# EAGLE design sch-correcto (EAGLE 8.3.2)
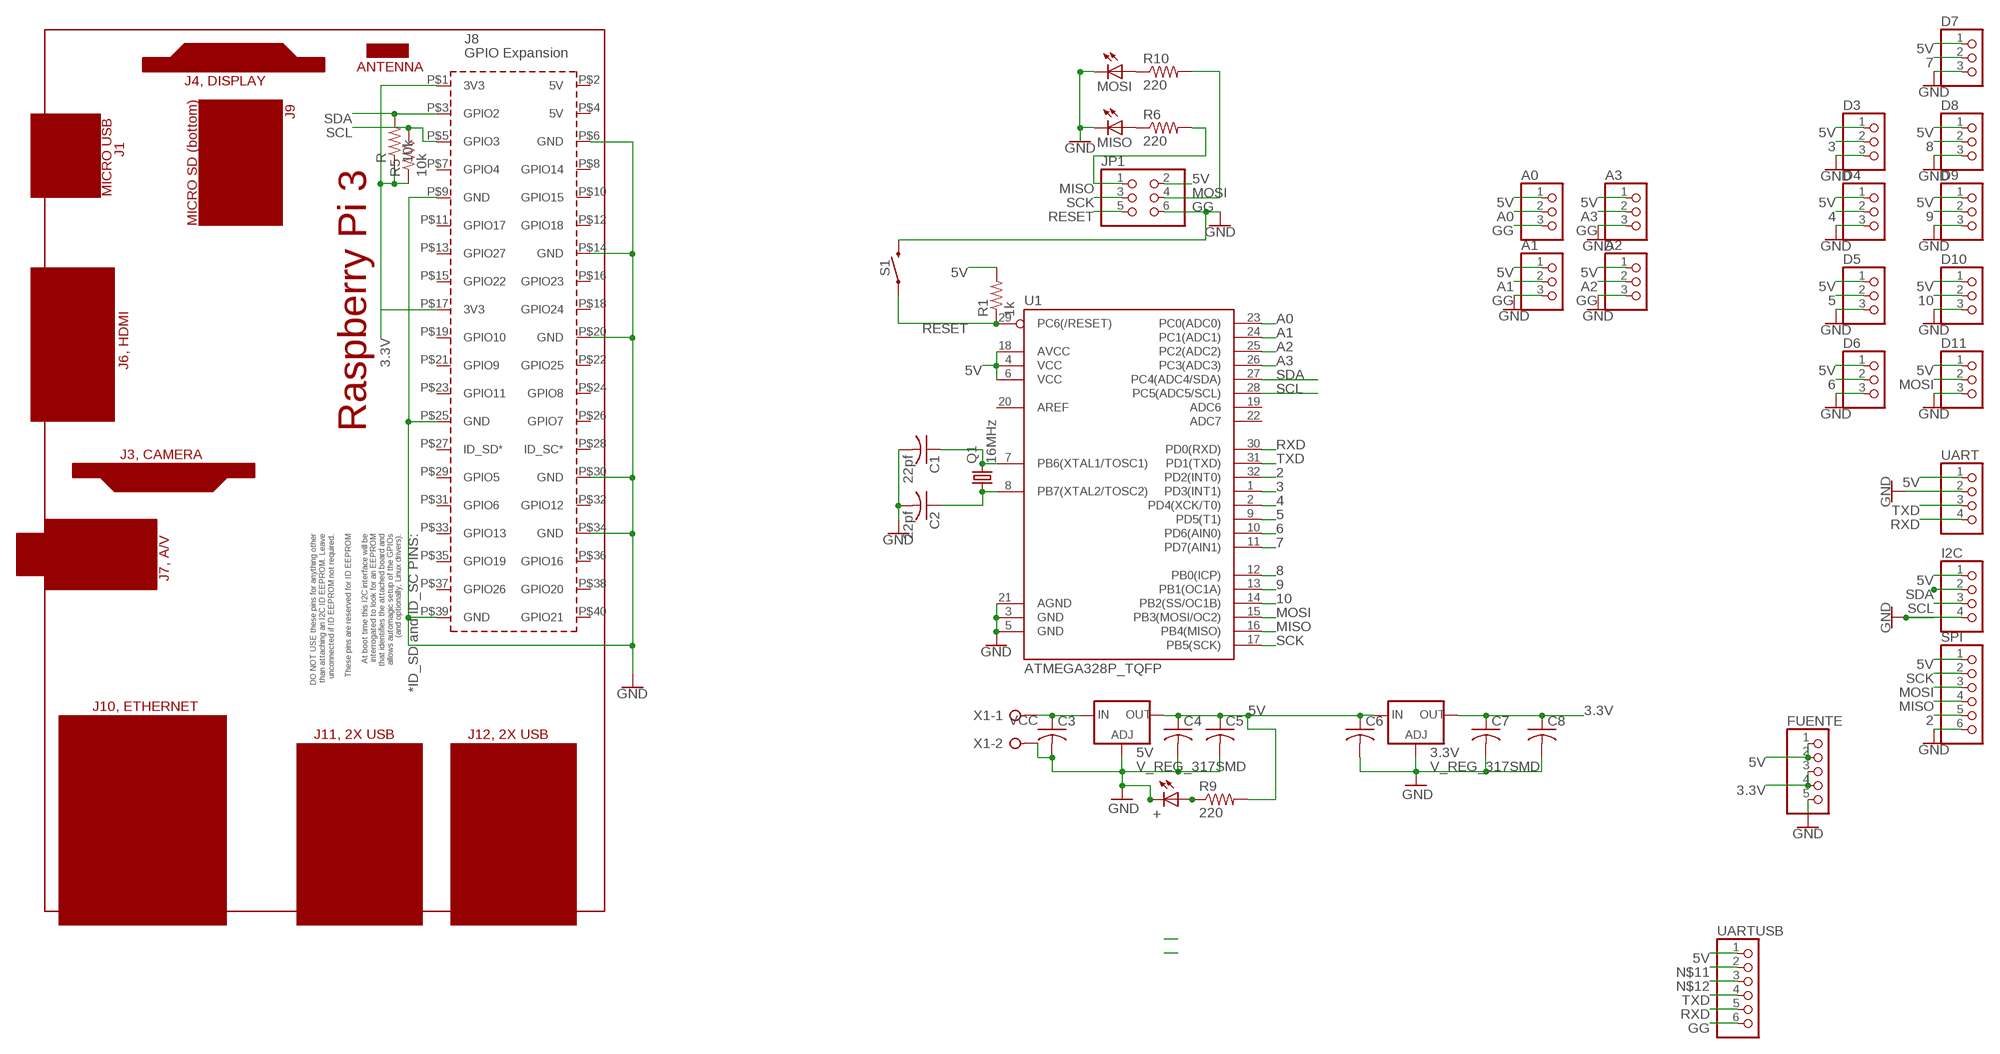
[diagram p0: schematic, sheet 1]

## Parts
3.3V  V_REG_317SMD  [SOT223]
5V  V_REG_317SMD  [SOT223]
+  LEDSML1206  [SML1206]
A0  PINHD-1X3  [1X03]
A1  PINHD-1X3  [1X03]
A2  PINHD-1X3  [1X03]
A3  PINHD-1X3  [1X03]
C1  22pf  C-USC1206  [C1206]
C2  22pf  C-USC1206  [C1206]
C3  C-USC1206  [C1206]
C4  C-USC1206  [C1206]
C5  C-USC1206  [C1206]
C6  C-USC1206  [C1206]
C7  C-USC1206  [C1206]
C8  C-USC1206  [C1206]
D3  PINHD-1X3  [1X03]
D4  PINHD-1X3  [1X03]
D5  PINHD-1X3  [1X03]
D6  PINHD-1X3  [1X03]
D7  PINHD-1X3  [1X03]
D8  PINHD-1X3  [1X03]
D9  PINHD-1X3  [1X03]
D10  PINHD-1X3  [1X03]
D11  PINHD-1X3  [1X03]
FUENTE  PINHD-1X5  [1X05]
I2C  PINHD-1X4  [1X04]
JP1  PINHD-2X3  [2X03]
MISO  LEDSML1206  [SML1206]
MOSI  LEDSML1206  [SML1206]
PCB1  RPI3  [RPI3]
Q1  16MHz  CRYSTALHC49UP  [HC49UP]
R  10k  R-US_M1206  [M1206]
R1  1k  R-US_M1206  [M1206]
R5  10k  R-US_M1206  [M1206]
R6  220  R-US_M1206  [M1206]
R9  220  R-US_M1206  [M1206]
R10  220  R-US_M1206  [M1206]
S1  MOMENTARY-SWITCH-SPST-SMD-6.2MM-TALL  [TACTILE_SWITCH_SMD_6.2MM_TALL]
SPI  PINHD-1X6  [1X06]
U1  ATMEGA328P_TQFP  [TQFP32-08]
UART  PINHD-1X4  [1X04]
UARTUSB  PINHD-1X6  [1X06]
X1  W237-02P  [W237-132]

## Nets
2: SPI.5 U1.32(PD2(INT0))
3: D3.2 U1.1(PD3(INT1))
3.3V: 3.3V.2(OUT) C7.1 C8.1 FUENTE.3 FUENTE.4 PCB1.P$1(3V3) PCB1.P$17(3V3) R5.1 R.1
4: D4.2 U1.2(PD4(XCK/T0))
5: D5.2 U1.9(PD5(T1))
5V: 3.3V.3(IN) 5V.2(OUT) A0.1 A1.1 A2.1 A3.1 C4.1 C5.1 C6.1 D3.1 D4.1 D5.1 D6.1 D7.1 D8.1 D9.1 D10.1 D11.1 FUENTE.1 FUENTE.2 I2C.1 JP1.2 R1.2 R9.2 SPI.1 U1.4(VCC) U1.6(VCC) U1.18(AVCC) UART.1 UARTUSB.1
6: D6.2 U1.10(PD6(AIN0))
7: D7.2 U1.11(PD7(AIN1))
8: D8.2 U1.12(PB0(ICP))
9: D9.2 U1.13(PB1(OC1A))
10: D10.2 U1.14(PB2(SS/OC1B))
A0: A0.2 U1.23(PC0(ADC0))
A1: A1.2 U1.24(PC1(ADC1))
A2: A2.2 U1.25(PC2(ADC2))
A3: A3.2 U1.26(PC3(ADC3))
GG: 3.3V.1(ADJ) 5V.1(ADJ) +.C A0.3 A1.3 A2.3 A3.3 C1.2 C2.2 C3.2 C4.2 C5.2 C6.2 C7.2 C8.2 D3.3 D4.3 D5.3 D6.3 D7.3 D8.3 D9.3 D10.3 D11.3 FUENTE.5 I2C.4 JP1.6 MISO.C MOSI.C PCB1.P$6(GND) PCB1.P$9(GND) PCB1.P$14(GND) PCB1.P$20(GND) PCB1.P$25(GND) PCB1.P$30(GND) PCB1.P$34(GND) PCB1.P$39(GND) S1.B2 SPI.6 U1.3(GND) U1.5(GND) U1.21(AGND) UART.2 UARTUSB.6 X1.2 ; supply symbol labelled GND
MISO: JP1.1 R6.2 SPI.4 U1.16(PB4(MISO))
MOSI: D11.2 JP1.4 R10.2 SPI.3 U1.15(PB3(MOSI/OC2))
N$1: C1.1 Q1.2 U1.7(PB6(XTAL1/TOSC1))
N$2: C2.1 Q1.1 U1.8(PB7(XTAL2/TOSC2))
N$4: +.A R9.1
N$8: MISO.A R6.1
N$9: MOSI.A R10.1
N$11: UARTUSB.2
N$12: UARTUSB.3
RESET: JP1.5 R1.1 S1.A2 U1.29(PC6(/RESET))
RXD: U1.30(PD0(RXD)) UART.4 UARTUSB.5
SCK: JP1.3 SPI.2 U1.17(PB5(SCK))
SCL: I2C.3 PCB1.P$5(GPIO3) R5.2 U1.28(PC5(ADC5/SCL))
SDA: I2C.2 PCB1.P$3(GPIO2) R.2 U1.27(PC4(ADC4/SDA))
TXD: U1.31(PD1(TXD)) UART.3 UARTUSB.4
VCC: 5V.3(IN) C3.1 X1.1
Unconnected: PCB1.P$2(5V) PCB1.P$4(5V) PCB1.P$7(GPIO4) PCB1.P$8(GPIO14) PCB1.P$10(GPIO15) PCB1.P$11(GPIO17) PCB1.P$12(GPIO18) PCB1.P$13(GPIO27) PCB1.P$15(GPIO22) PCB1.P$16(GPIO23) PCB1.P$18(GPIO24) PCB1.P$19(GPIO10) PCB1.P$21(GPIO9) PCB1.P$22(GPIO25) PCB1.P$23(GPIO11) PCB1.P$24(GPIO8) PCB1.P$26(GPIO7) PCB1.P$27(ID_SD*) PCB1.P$28(ID_SC*) PCB1.P$29(GPIO5) PCB1.P$31(GPIO6) PCB1.P$32(GPIO12) PCB1.P$33(GPIO13) PCB1.P$35(GPIO19) PCB1.P$36(GPIO16) PCB1.P$37(GPIO26) PCB1.P$38(GPIO20) PCB1.P$40(GPIO21) U1.19(ADC6) U1.20(AREF) U1.22(ADC7)

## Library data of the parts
3.3V 5V = SparkFun-IC-Power:V_REG_317: Voltage Regulator Standard LM317 adjustable voltage regulator. AOI (Adjust Output Input). Google 'LM317 Calculator' for easy to use app to get the two resistor values needed. 240/720 for 5V output. 240/390 for 3.3V output. Spark Fun Electronics SKU : COM-00527
+ MISO MOSI = led:LED: LED
A0 A1-A3 D3-D11 = pinhead:PINHD-1X3: PIN HEADER
C1 C2 = rcl:C-US: CAPACITOR, American symbol
C3-C8 = resistor:C-US: CAPACITOR, American symbol
FUENTE = pinhead:PINHD-1X5: PIN HEADER
I2C UART = pinhead:PINHD-1X4: PIN HEADER
JP1 = pinhead:PINHD-2X3: PIN HEADER
PCB1 = e14_Rpi3_RevA:RPI3: Device for Raspberry Pi 3 board created by Dave Young for www.element14.com More information and support community is available at https://www.element14.com/community/community/raspberry-pi
Q1 = crystal:CRYSTAL: CRYSTAL; OC_FARNELL: unknown; OC_NEWARK: unknown
R R1 R5 R6 R9 R10 = resistor:R-US_: RESISTOR, American symbol
S1 = SparkFun-Switches:MOMENTARY-SWITCH-SPST: Momentary Switch (Pushbutton) - SPST; PROD_ID: SWCH-11966; SF_SKU: COM-12992
SPI UARTUSB = pinhead:PINHD-1X6: PIN HEADER
U1 = SparkFun-DigitalIC:ATMEGA328P_TQFP; PROD_ID: IC-09069
X1 = con-wago-508:W237-02P: WAGO SREW CLAMP; OC_FARNELL: unknown; OC_NEWARK: unknown

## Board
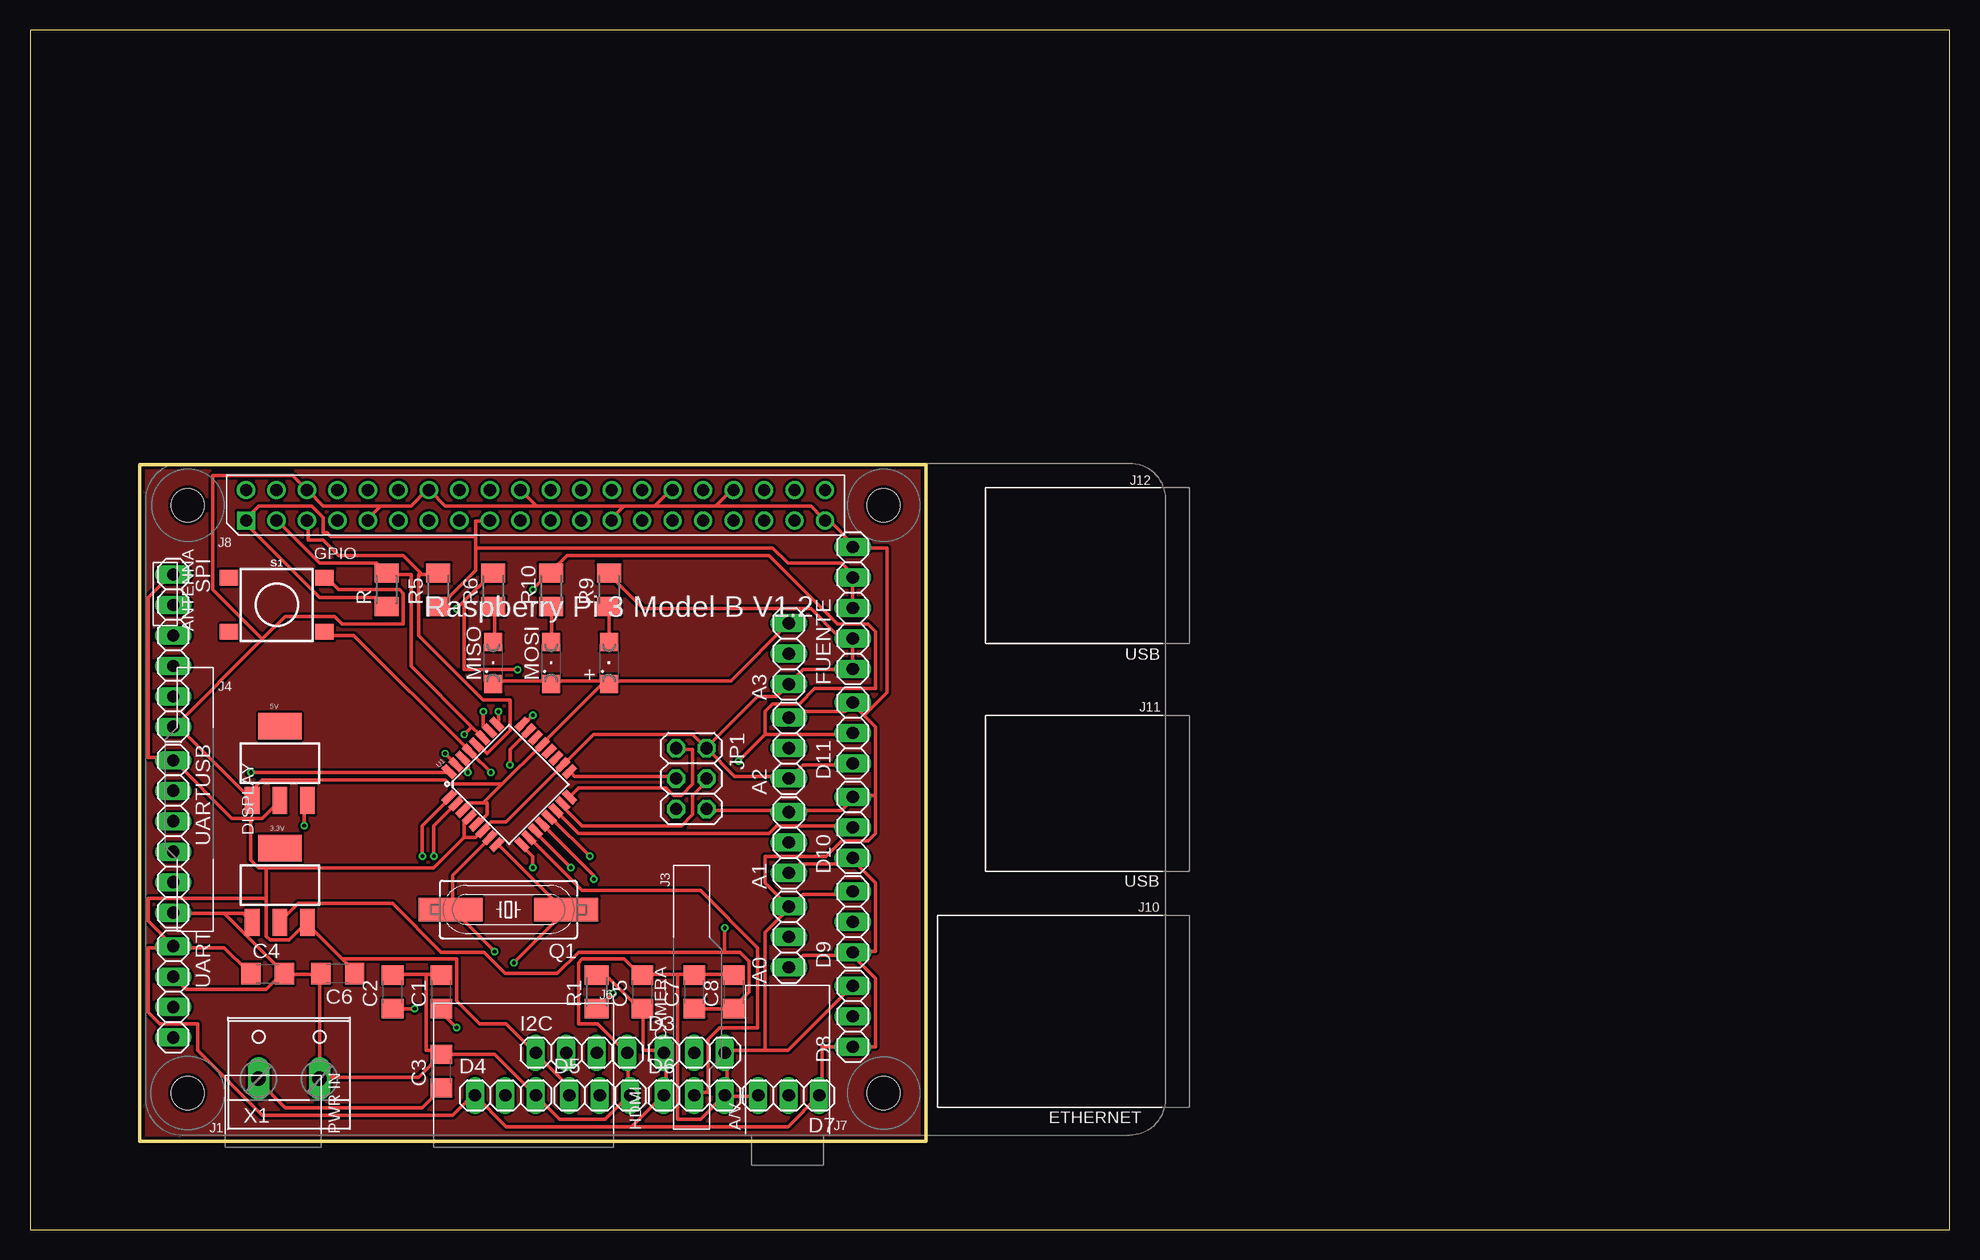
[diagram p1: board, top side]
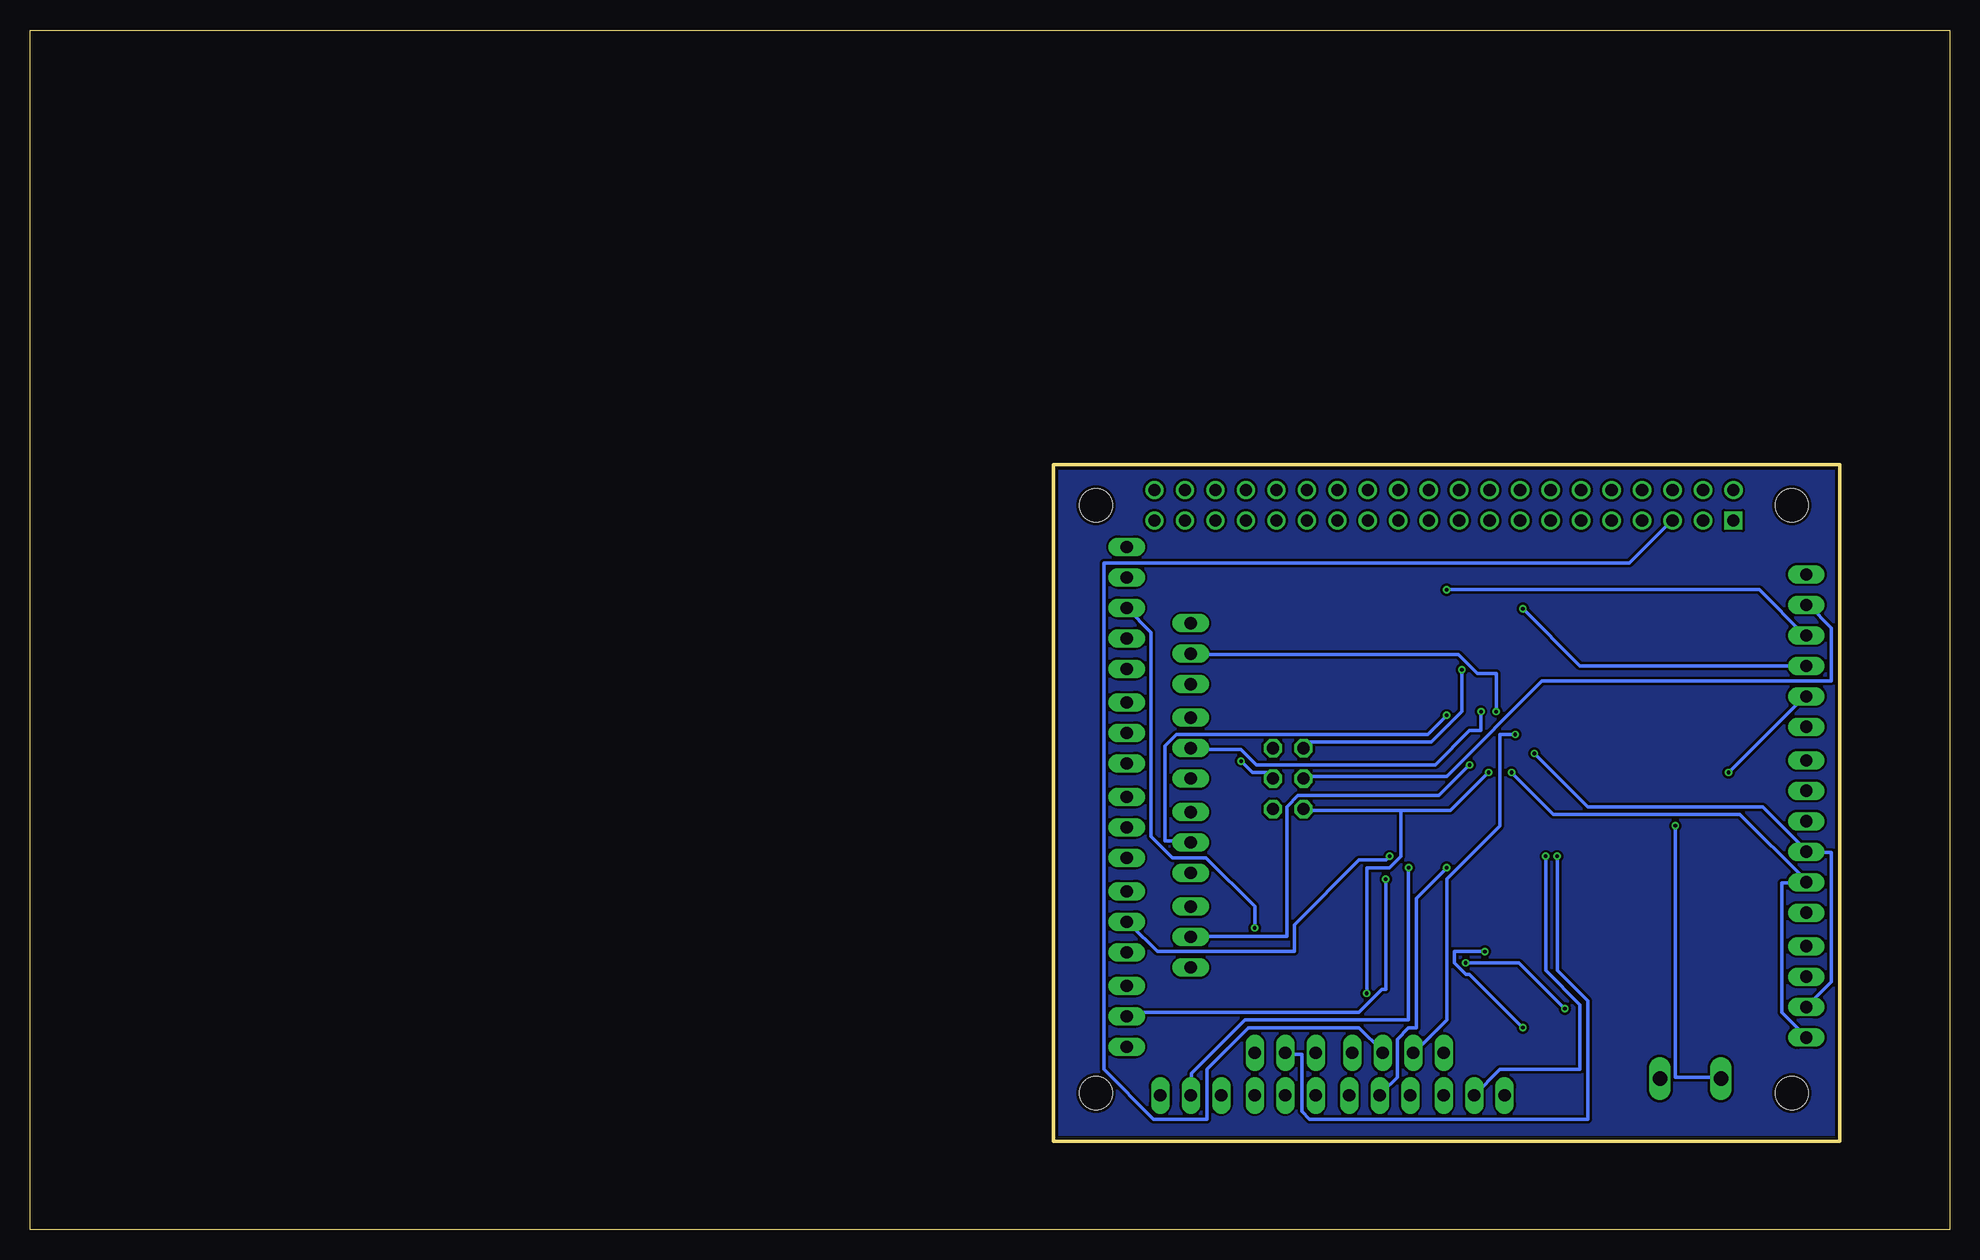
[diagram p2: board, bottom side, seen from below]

Size 160 x 100 mm. Coordinates in mm from the lower left corner, seen from the top.
Outline: 0,0 160,0 160,100 0,100 0,0
Outline: 9.14,7.37 74.68,7.37 74.68,63.75 9.14,63.75 9.14,7.37
Copper layers (1*16): Top 0.035mm / dielectric 1.5mm / Bottom 0.035mm
Design rules "RYSPEE_2layer_DRU *": minimum track width 12mil, minimum drill 12mil, track to track 8mil, track to pad 8mil, pad to pad 8mil, via to via 8mil, smd to smd 8mil, copper to edge 10mil, drill to drill 10mil, minimum pad ring 10mil, minimum via ring 6mil, stop-mask expansion 2mil, vias tented up to drill 100mil, thermal gap 10mil

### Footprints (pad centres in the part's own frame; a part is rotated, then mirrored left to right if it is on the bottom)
SOT223 = smd 1.219 x 2.235: 1 -2.311,-3.099; 2 0,-3.099; 3 2.311,-3.099 | smd 3.6 x 2.2: 4 0,3.099
SML1206 = smd 1.5 x 1.5: A 1.75,0; C -1.75,0
1X03 = drill 1.016 long: 1 -2.54,0; 2 0,0; 3 2.54,0
C1206 = smd 1.6 x 1.8: 1 -1.4,0; 2 1.4,0
1X05 = drill 1.016 long: 1 -5.08,0; 2 -2.54,0; 3 0,0; 4 2.54,0; 5 5.08,0
1X04 = drill 1.016 long: 1 -3.81,0; 2 -1.27,0; 3 1.27,0; 4 3.81,0
2X03 = drill 1.016 octagon: 1 -2.54,-1.27; 2 -2.54,1.27; 3 0,-1.27; 4 0,1.27; 5 2.54,-1.27; 6 2.54,1.27
RPI3 = drill 1.016 square: P$1 8.37,51.23 | drill 1.016: P$2 8.357,53.772; P$3 10.897,51.232; P$4 10.897,53.772; P$5 13.437,51.232; P$6 13.437,53.772; P$7 15.977,51.232; P$8 15.977,53.772; P$9 18.517,51.232; P$10 18.517,53.772; P$11 21.057,51.232; P$12 21.057,53.772; P$13 23.597,51.232; P$14 23.597,53.772; P$15 26.137,51.232; P$16 26.137,53.772; P$17 28.677,51.232; P$18 28.677,53.772; P$19 31.217,51.232; P$20 31.217,53.772; P$21 33.757,51.232; P$22 33.757,53.772; P$23 36.297,51.232; P$24 36.297,53.772; P$25 38.837,51.232; P$26 38.837,53.772; P$27 41.377,51.232; P$28 41.377,53.772; P$29 43.917,51.232; P$30 43.917,53.772; P$31 46.457,51.232; P$32 46.457,53.772; P$33 48.997,51.232; P$34 48.997,53.772; P$35 51.537,51.232; P$36 51.537,53.772; P$37 54.077,51.232; P$38 54.077,53.772; P$39 56.617,51.232; P$40 56.617,53.772 | hole 2.75: 3.5,3.5; 61.5,3.5; 3.5,52.5; 61.5,52.5
HC49UP = smd 5.334 x 1.93: 1 -4.826,0; 2 4.826,0
M1206 = smd 1.6 x 2: 1 -1.4,0; 2 1.4,0
TACTILE_SWITCH_SMD_6.2MM_TALL = smd 1.55 x 1.3: A1 -3.975,-2.25; A2 3.975,-2.25; B1 -3.975,2.25; B2 3.975,2.25
1X06 = drill 1.016 long: 1 -6.35,0; 2 -3.81,0; 3 -1.27,0; 4 1.27,0; 5 3.81,0; 6 6.35,0
TQFP32-08 = smd 1.27 x 0.559: 1 -4.293,2.8; 2 -4.293,2; 3 -4.293,1.2; 4 -4.293,0.4; 5 -4.293,-0.4; 6 -4.293,-1.2; 7 -4.293,-2; 8 -4.293,-2.8; 17 4.293,-2.8; 18 4.293,-2; 19 4.293,-1.2; 20 4.293,-0.4; 21 4.293,0.4; 22 4.293,1.2; 23 4.293,2; 24 4.293,2.8 | smd 0.559 x 1.27: 9 -2.8,-4.293; 10 -2,-4.293; 11 -1.2,-4.293; 12 -0.4,-4.293; 13 0.4,-4.293; 14 1.2,-4.293; 15 2,-4.293; 16 2.8,-4.293; 25 2.8,4.293; 26 2,4.293; 27 1.2,4.293; 28 0.4,4.293; 29 -0.4,4.293; 30 -1.2,4.293; 31 -2,4.293; 32 -2.8,4.293
W237-132 = drill 1.194 long: 1 -2.54,-0.635; 2 2.54,-0.635

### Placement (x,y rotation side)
3.3V  20.83,28.7 0 top
5V  20.83,38.86 0 top
+  48.26,47.24 90 top
A0  63.25,24.38 90 top
A1  63.25,32.26 90 top
A2  63.25,40.13 90 top
A3  63.25,48.01 90 top
C1  34.29,19.81 90 top
C2  30.23,19.81 90 top
C3  34.29,13.21 90 top
C4  19.81,21.34 0 top
C5  51.05,19.81 90 top
C6  25.65,21.34 180 top
C7  55.37,19.81 90 top
C8  58.67,19.81 90 top
D3  55.37,14.73 0 top
D4  39.62,11.18 0 top
D5  47.5,11.18 0 top
D6  55.37,11.18 0 top
D7  63.25,11.18 180 top
D8  68.58,17.78 90 top
D9  68.58,25.65 90 top
D10  68.58,33.53 90 top
D11  68.58,41.4 90 top
FUENTE  68.58,51.82 90 top
I2C  45.97,14.73 0 top
JP1  55.12,37.59 270 top
MISO  38.61,47.24 90 top
MOSI  43.43,47.24 90 top
PCB1  9.65,7.87 0 top
Q1  39.88,26.67 180 top
R  29.72,53.34 90 top
R1  47.24,19.81 90 top
R5  34.04,53.34 90 top
R6  38.61,53.34 90 top
R9  48.26,53.34 90 top
R10  43.43,53.34 90 top
S1  20.57,52.07 0 top
SPI  11.94,48.26 270 top
U1  39.95,37.11 45 top
UART  11.94,19.81 270 top
UARTUSB  11.94,32.77 270 top
X1  21.59,13.21 0 top

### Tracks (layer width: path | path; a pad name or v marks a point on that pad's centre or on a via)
2  (via drill 0.3)
  Top 0.305: v18.41,38.1 34.92,38.1 U1.32
  Bottom 0.305: v18.41,38.1 12.06,44.45 SPI.5
3  (via drill 0.3)
  Top 0.305: v32.7,31.11 32.7,33.66 34.92,35.88 U1.1
  Bottom 0.305: v32.7,31.11 32.7,21.59 30.16,19.05 30.16,9.21 53.34,9.21 53.98,9.84 53.98,14.61 55.24,14.61 D3.2
3.3V  (via drill 0.3)
  Top 0.305: C7.1 55.56,18.41 58.42,18.41 C8.1 58.67,18.54 59.94,19.81 59.94,22.35 59.18,23.11 57.91,23.11 | R.1 29.53,52.07 28.89,52.7 24.13,52.7 17.78,59.05 PCB1.P$1 18.1,59.37 19.05,60.33 23.5,60.33 24.45,59.37 24.45,58.1 24.77,58.1 25.08,57.78 37.15,57.78 | FUENTE.3 FUENTE.4 68.58,54.61 67.63,55.56 63.18,55.56 61.91,56.83 37.15,56.83 | 37.15,57.78 37.15,59.05 38.1,59.05 PCB1.P$17 | 37.15,57.78 37.15,56.83 | 37.15,56.83 37.15,54.93 34.29,52.07 R5.1 | 57.91,23.11 45.72,23.11 43.94,21.34 39.62,21.34 37.85,23.11 34.29,23.11 30.23,27.18 22.35,27.18 20.83,25.65 3.3V.2 | v57.91,25.15 57.91,23.11
  Bottom 0.305: v57.91,25.15 57.91,26.92 61.98,30.99 64.77,30.99 66.55,32.77 66.55,49.78 FUENTE.3
4  (via drill 0.3)
  Top 0.305: v33.66,31.11 33.66,33.66 35.24,35.24 U1.2
  Bottom 0.305: v33.66,31.11 33.66,21.59 30.8,18.73 30.8,13.34 37.47,13.34 D4.2
5  (via drill 0.3)
  Top 0.305: v41.91,30.16 41.91,31.11 40.96,32.07 U1.9
  Bottom 0.305: v41.91,30.16 44.45,27.62 44.45,16.83 45.09,16.83 46.04,15.88 46.04,12.7 47.31,11.43 D5.2
5V
  Top 0.305: 68.58,30.8 68.26,30.48 64.14,30.48 63.5,29.84 A1.1 | 68.58,22.86 64.45,22.86 63.5,21.91 A0.1 | 68.58,22.86 70.48,20.95 70.48,15.24 D8.1 66.04,15.24 66.04,11.43 D7.1 63.18,8.57 50.16,8.57 | 68.58,22.86 D9.1 68.58,23.18 70.48,23.18 70.48,28.89 68.58,30.8 | 68.58,30.8 D10.1 | R1.2 47.31,20.95 48.26,20.95 50.8,18.41 C5.1 51.12,18.1 51.12,14.92 52.7,14.92 D3.1 53.02,14.61 53.02,11.43 D6.1 52.7,11.11 50.16,8.57 | 50.16,8.57 39.69,8.57 D4.1 36.83,11.11 35.24,9.53 19.37,9.53 13.97,14.92 13.97,17.14 10.79,17.14 9.84,18.1 9.84,23.5 11.75,23.5 UART.1 | R9.2 48.26,54.61 51.12,51.75 65.09,51.75 67.31,49.53 68.58,49.53 FUENTE.2 FUENTE.1 68.58,46.67 64.45,46.67 A3.1 62.23,44.45 60.64,44.45 56.52,40.32 JP1.2 | 36.2,32.7 36.2,33.97 36.51,34.29 U1.4 | 36.2,32.7 37.15,32.7 37.47,33.02 U1.6 37.78,33.34 38.42,33.97 39.69,33.97 44.45,38.73 | D11.1 68.58,38.73 64.45,38.73 63.5,37.78 A2.1 63.18,37.78 58.74,37.78 JP1.2 | 44.45,38.73 46.99,41.27 55.24,41.27 JP1.2 | 44.45,38.73 U1.18 | C4.1 18.1,21.59 16.19,23.5 12.06,23.5 UART.1 | D5.1 44.77,11.43 44.77,12.06 42.23,14.61 I2C.1 41.91,14.92 39.69,17.14 37.47,17.14 35.56,19.05 35.56,22.54 26.04,22.54 | 26.04,22.54 23.18,25.4 3.3V.3 22.86,25.4 21.59,24.13 20,24.13 19.68,24.45 19.68,27.62 | 26.04,22.54 26.99,21.59 C6.1 | 18.41,34.29 16.83,34.29 12.06,39.05 UARTUSB.1 11.75,39.37 9.84,39.37 9.84,52.7 11.75,54.61 SPI.1 | 18.41,34.29 19.37,34.29 20.64,35.56 5V.2 | 19.68,30.16 19.68,27.62 | 19.68,30.16 19.05,30.16 18.41,30.8 18.41,34.29 | UART.1 9.84,25.72 9.84,27.62 19.68,27.62 | 36.2,32.7 33.66,30.16 19.68,30.16
6
  Top 0.305: U1.10 41.59,32.7 46.04,28.26 55.88,28.26 60.64,23.5 60.64,16.83 57.47,16.83 56.52,15.88 56.52,11.43 55.56,11.43 D6.2
7  (via drill 0.3)
  Top 0.305: v45.09,30.16 42.23,33.02 U1.11
  Bottom 0.305: v45.09,30.16 45.09,17.46 58.74,17.46 63.18,13.02 63.18,11.43 D7.2
8  (via drill 0.3)
  Top 0.305: v46.99,29.21 46.99,29.53 42.86,33.66 U1.12
  Bottom 0.305: v46.99,29.21 46.99,20 47.31,20 49.21,18.1 68.26,18.1 D8.2
9  (via drill 0.3)
  Top 0.305: v46.67,31.11 43.5,34.29 U1.13
  Bottom 0.305: v46.67,31.11 46.99,30.8 49.21,30.8 54.61,25.4 54.61,23.18 66.04,23.18 68.26,25.4 68.58,25.4 D9.2
10
  Top 0.305: U1.14 43.81,34.92 45.72,33.02 61.59,33.02 62.23,33.66 68.58,33.66 D10.2
A0  (via drill 0.3)
  Top 0.305: v40.01,38.73 40.01,40.01 41.27,41.27 U1.23
  Bottom 0.305: v40.01,38.73 42.55,36.2 54.29,36.2 55.24,35.24 55.24,24.45 63.18,24.45 A0.2
A1  (via drill 0.3)
  Top 0.305: v41.91,42.86 41.27,42.23 U1.24
  Bottom 0.305: v41.91,42.86 43.5,41.27 64.45,41.27 65.41,40.32 65.41,32.38 63.5,32.38 A1.2
A2  (via drill 0.3)
  Top 0.305: v39.05,43.18 39.05,42.23 U1.25
  Bottom 0.305: v39.05,43.18 39.05,41.59 40.01,41.59 42.86,38.73 57.78,38.73 59.05,40.01 63.18,40.01 A2.2
A3  (via drill 0.3)
  Top 0.305: v37.78,43.18 37.78,41.91 38.1,41.59 U1.26
  Bottom 0.305: v37.78,43.18 37.78,46.35 39.37,46.35 40.96,47.94 63.18,47.94 A3.2
GG
  Top 0.305: A0.3 63.5,26.99 64.45,27.94 68.58,27.94 D9.3 | 53.98,21.27 55.24,21.27 C7.2 55.56,21.27 58.42,21.27 C8.2 | 53.98,21.27 51.12,21.27 C5.2 50.8,21.27 49.53,22.54 46.04,22.54 45.72,22.23 45.72,17.14 47.31,17.14 49.53,14.92 I2C.4 49.85,14.61 49.85,11.43 D5.3 49.85,11.11 47.94,9.21 44.13,9.21 D4.3 38.73,14.61 C3.2 | D6.3 58.1,11.11 60.64,11.11 D7.3 | D6.3 58.1,11.43 58.1,14.61 D3.3 58.1,14.92 61.28,14.92 | D8.3 63.18,14.92 61.28,14.92 | 53.98,21.27 53.98,9.21 55.88,9.21 57.78,11.11 D6.3 | 61.28,14.92 61.28,24.77 63.18,26.67 A0.3 | 24.13,21.27 21.27,21.27 C4.2 | 16.19,26.35 12.06,26.35 UARTUSB.6 | 16.19,26.35 17.78,26.35 18.41,25.72 3.3V.1 | 16.19,26.35 20.95,21.59 C4.2 | UART.2 13.02,20 19.68,20 20.95,21.27 C4.2 | 33.02,21.27 34.29,21.27 C1.2 | 33.02,21.27 30.48,21.27 C2.2 | C3.2 32.38,12.7 24.13,12.7 | C3.2 34.29,14.92 33.02,14.92 33.02,21.27 | 24.13,12.7 24.13,21.27 | 24.13,21.27 C6.2 | 24.13,12.7 X1.2 | 12.06,41.91 19.37,49.21 | 19.37,49.21 21.27,51.12 25.4,51.12 26.04,50.48 31.11,50.48 31.11,53.02 30.8,53.34 25.72,53.34 24.77,54.29 S1.B2 | 18.1,36.2 12.38,41.91 12.06,41.91 | 18.1,36.2 18.41,35.88 5V.1 18.1,36.2 | 12.06,41.91 SPI.6 | 37.78,35.56 36.51,35.56 36.2,35.24 U1.3 | 37.78,35.56 38.1,35.56 38.1,34.61 37.47,33.97 U1.5 | 37.78,35.56 39.37,37.15 | 39.37,37.15 42.55,40.32 U1.21 42.86,40.64 47.94,45.72 | MISO.C 38.73,45.72 43.18,45.72 MOSI.C 43.5,45.72 47.94,45.72 | 47.94,45.72 48.26,45.72 | A3.3 58.42,45.72 48.26,45.72 | 48.26,45.72 +.C 47.94,45.72 | 18.1,36.2 19.37,37.47 34.61,37.47 34.92,37.15 39.37,37.15 | 68.58,43.81 67.94,43.18 63.82,43.18 63.5,42.86 A2.3 | JP1.6 56.52,34.92 63.18,34.92 A1.3 63.5,34.92 67.63,34.92 68.58,35.88 D10.3 68.58,36.2 70.48,36.2
  Top 0.305: 69.53,42.86 70.48,41.91 70.48,36.2 | 69.53,42.86 68.58,43.81 | 68.58,43.81 D11.3 | 29.21,60.33 28.26,59.37 PCB1.P$9 | 29.21,60.33 31.75,60.33 33.02,61.59 PCB1.P$14 33.34,61.59 34.61,60.33 42.23,60.33 | 29.21,60.33 24.45,60.33 23.18,61.59 PCB1.P$6 22.86,61.91 21.91,62.87 15.24,62.87 15.24,53.34 19.37,49.21 | 49.53,60.33 48.58,59.37 PCB1.P$25 | 52.07,60.33 49.53,60.33 | 52.07,60.33 53.34,61.59 PCB1.P$30 | 42.23,60.33 40.96,61.59 PCB1.P$20 | 49.53,60.33 42.23,60.33 | 57.15,60.33 58.42,61.59 PCB1.P$34 | 52.07,60.33 57.15,60.33 | 57.15,60.33 65.09,60.33 66.04,59.37 PCB1.P$39 66.36,59.05 66.67,59.05 68.58,57.15 FUENTE.5 68.58,56.83 71.44,56.83 71.44,44.77 69.53,42.86 | A0.3 61.28,28.89 61.28,31.11 66.36,31.11 67.63,32.38 69.85,32.38 70.48,33.02 70.48,36.2
GND
  pour Top: 9.4,7.62 74.42,7.62 74.42,63.5 9.4,63.5
  pour Bottom: 9.4,7.62 74.42,7.62 74.42,63.5 9.4,63.5
MISO  (via drill 0.3)
  Top 0.305: U1.16 45.09,36.2 45.72,36.83 53.02,36.83 53.66,36.2 54.29,36.2 55.24,37.15 55.24,40.01 53.98,40.01 JP1.1 | v35.56,51.75 36.2,52.39 | 36.2,52.39 38.42,54.61 R6.2 | v40.64,46.67 36.2,46.67 36.2,52.39
  Bottom 0.305: v35.56,51.75 30.8,46.99 SPI.4 | JP1.1 53.34,40.64 43.18,40.64 40.64,43.18 v40.64,46.67
MOSI  (via drill 0.3)
  Top 0.305: U1.15 44.45,35.24 46.04,33.66 54.29,33.66 55.24,34.61 55.24,36.2 56.52,37.47 JP1.4 | 61.28,41.27 61.28,43.18 61.91,43.81 64.14,43.81 65.41,45.09 70.48,45.09 70.48,49.85 69.85,50.48 67.31,50.48 61.59,56.2 44.77,56.2 43.5,54.93 R10.2 43.18,54.61 v41.91,53.34 | 61.28,41.27 68.58,41.27 D11.2 | 61.28,41.27 v59.05,39.05
  Bottom 0.305: v41.91,53.34 15.88,53.34 12.06,49.53 SPI.3 | v59.05,39.05 58.1,38.1 56.83,38.1 56.52,37.78 JP1.4
N$1  (via drill 0.3)
  Top 0.305: 35.24,26.67 35.24,29.53 38.1,32.38 U1.7 | v35.56,16.83 34.29,18.1 C1.1 | 35.24,26.67 v38.73,23.18 | 35.24,26.67 Q1.2
  Bottom 0.305: v35.56,16.83 40.01,21.27 40.32,21.27 41.27,22.23 41.27,23.18 v38.73,23.18
N$2  (via drill 0.3)
  Top 0.305: 44.45,26.67 39.05,32.07 U1.8 | v32.07,18.41 30.48,18.41 C2.1 | v40.32,22.23 44.45,26.35 44.45,26.67 | 44.45,26.67 Q1.1
  Bottom 0.305: v32.07,18.41 35.88,22.23 v40.32,22.23
N$4
  Top 0.305: R9.1 +.A
N$8
  Top 0.305: MISO.A 38.73,49.21 38.73,51.75 R6.1
N$9
  Top 0.305: MOSI.A 43.5,49.21 43.5,51.75 R10.1
RESET  (via drill 0.3)
  Top 0.305: S1.A2 24.77,49.53 26.99,49.53 36.51,40.01 U1.29 36.83,39.69 v38.42,38.1 | v48.58,19.68 47.31,18.41 R1.1
  Bottom 0.305: v48.58,19.68 48.58,30.16 46.67,30.16 45.72,31.11 45.72,34.92 | 45.72,34.92 53.66,34.92 JP1.5 | v38.42,38.1 41.59,34.92 45.72,34.92
RXD  (via drill 0.3)
  Top 0.305: v36.51,38.1 36.51,38.73 36.2,39.05 U1.30
  Bottom 0.305: v36.51,38.1 33.02,34.61 17.46,34.61 12.06,29.21 UARTUSB.5 12.06,28.89 13.97,28.89 13.97,18.1 12.06,16.19 UART.4
SCK
  Top 0.305: U1.17 45.09,38.1 45.4,37.78 53.66,37.78 JP1.3
  Bottom 0.305: SPI.2 11.75,52.07 9.84,50.16 9.84,45.72 33.97,45.72 41.91,37.78 53.66,37.78 JP1.3
SCL
  Top 0.305: 32.7,54.61 33.97,54.61 R5.2 | 32.7,54.61 32.38,54.61 32.38,49.53 37.78,44.13 40.01,44.13 40.01,41.59 38.1,39.69 37.47,40.32 U1.28 | 32.7,54.61 31.11,56.2 25.72,56.2 24.45,57.47 23.18,57.47 23.18,59.05 PCB1.P$5
  Bottom 0.305: I2C.3 47.31,14.92 49.21,16.83 58.42,16.83 61.91,13.34 61.91,9.21 66.36,9.21 70.48,13.34 70.48,55.56 26.67,55.56 23.18,59.05 PCB1.P$5
SDA  (via drill 0.3)
  Top 0.305: 36.83,41.91 31.75,46.99 31.75,54.61 29.84,54.61 R.2 29.53,54.93 28.89,55.56 24.13,55.56 20.64,59.05 PCB1.P$3 | 36.83,41.91 37.47,41.27 U1.27 | 36.83,41.91 v36.2,41.27
  Bottom 0.305: v36.2,41.27 37.47,41.27 37.47,33.66 41.91,29.21 41.91,17.46 44.45,14.92 I2C.2
TXD  (via drill 0.3)
  Top 0.305: v34.61,39.69 35.24,39.05 U1.31
  Bottom 0.305: v34.61,39.69 30.16,35.24 15.56,35.24 12.06,31.75 UARTUSB.4 11.75,31.43 9.84,31.43 9.84,20.64 UART.3
VCC  (via drill 0.3)
  Top 0.305: C3.1 34.29,11.75 32.7,10.16 21.27,10.16 19.05,12.38 X1.1 | v22.86,33.66 22.86,35.56 5V.3
  Bottom 0.305: v22.86,33.66 22.86,12.7 19.05,12.7 X1.1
